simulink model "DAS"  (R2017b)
settings: Solver=FixedStepDiscrete  StartTime=0.0  StopTime=10.0  FixedStep=0.01  RelTol=1e-3  EnableMultiTasking=on
undefined symbols (not defined in the file): CcDAS_ACModeCurtLim_A, CcDAS_ACModeCurtTiLim_ms, CcDAS_BMSOperationConfirmTi_ms, CcDAS_CellMaxTempLim1_C, CcDAS_CellMaxTempLim2_C, CcDAS_CellMaxTempLim3_C, CcDAS_CellMaxTempLim4_C, CcDAS_CellMinTempHiLim_C, CcDAS_CellMinTempLowLim_C, CcDAS_CellMinTempMidLim_C, CcDAS_CellTempDiffLim_C, CcDAS_DCModeCurtTiLim_ms, CcDAS_HVSafetyNVMStoreTi_ms, CcDAS_OCVSOCDiffLim1_numb, CcDAS_OCVSOCDiffLim2_numb, CcDAS_PackCurrLim_A, CcDAS_SOCHighLim_numb, CcDAS_SOCLowerLim_numb, CcDAS_SOHLowerLim_numb, CcDAS_SOHLowerLimSale_numb, DAS_MIN2MS_NUMB, DAS_RUNTIME100_MS, DAS_RUNTIME10_MS, DAS_STATSTIMEMAX_MIN, DAS_STATSTIMEMIN_MIN, DAS_STATSTIMESMAX_NUMB, DAS_STATSTIMESMIN_NUMB, DAS_TIMESONE_NUMB, Enum_CTCCtrCtlConnMode
libraries: AIWAYS_Powertrain_BMS_lib x268
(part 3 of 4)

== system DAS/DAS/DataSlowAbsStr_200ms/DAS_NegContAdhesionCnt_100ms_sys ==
  GbISP_TFNegCloseFlt_flg : Inport
  EdgeRising : AIWAYS_Powertrain_BMS_lib/Logical Operators/EdgeRising
  TimesAddition : Subsystem  TreatAsAtomicUnit=on
  GcDAS_NegContAdhesionCnt_numb : Outport
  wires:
  GbISP_TFNegCloseFlt_flg/1 -> EdgeRising/1
  EdgeRising/1 -> TimesAddition/Enable
  TimesAddition/1(GcDAS_NegContAdhesionCnt_numb) -> GcDAS_NegContAdhesionCnt_numb/1

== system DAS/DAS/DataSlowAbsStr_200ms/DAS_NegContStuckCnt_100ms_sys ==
  GbISP_TFNegOpenFlt_flg : Inport
  EdgeRising : AIWAYS_Powertrain_BMS_lib/Logical Operators/EdgeRising
  TimesAddition : Subsystem  TreatAsAtomicUnit=on
  GcDAS_NegContStuckCnt_numb : Outport
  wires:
  GbISP_TFNegOpenFlt_flg/1 -> EdgeRising/1
  EdgeRising/1 -> TimesAddition/Enable
  TimesAddition/1(GcDAS_NegContStuckCnt_numb) -> GcDAS_NegContStuckCnt_numb/1

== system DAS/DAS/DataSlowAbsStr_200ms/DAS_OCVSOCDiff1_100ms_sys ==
  GcSOC_MaxCellSOC_pct : Inport
  GcSOC_MinCellSOC_pct : Inport  Port=2
  Comparison1 : RelationalOperator  OutDataTypeStr=boolean
  Comparison3 : RelationalOperator  Operator=>  OutDataTypeStr=boolean
  Constant1 : Constant  Value=CcDAS_OCVSOCDiffLim1_numb
  Constant2 : Constant  Value=CcDAS_OCVSOCDiffLim2_numb
  Logical : Logic  OutDataTypeStr=boolean
  OperationTimeCalc : Subsystem
  Sum1 : Sum  Inputs=+-  OutDataTypeStr=Inherit: Inherit via back propagation  RndMeth=Zero
  GcDAS_OCVSOCDiffTi1_min : Outport
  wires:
  OperationTimeCalc/1(GcDAS_OCVSOCDiffTi1_min) -> GcDAS_OCVSOCDiffTi1_min/1
  GcSOC_MaxCellSOC_pct/1 -> Sum1/1
  GcSOC_MinCellSOC_pct/1 -> Sum1/2
  Sum1/1 -> Comparison1/2, Comparison3/1
  Constant1/1 -> Comparison3/2
  Constant2/1 -> Comparison1/1
  Comparison1/1 -> Logical/1
  Comparison3/1 -> Logical/2
  Logical/1 -> OperationTimeCalc/Enable

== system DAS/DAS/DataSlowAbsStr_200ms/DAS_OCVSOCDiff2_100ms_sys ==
  GcSOC_MaxCellSOC_pct : Inport
  GcSOC_MinCellSOC_pct : Inport  Port=2
  Comparison3 : RelationalOperator  Operator=>  OutDataTypeStr=boolean
  Constant1 : Constant  Value=CcDAS_OCVSOCDiffLim2_numb
  OperationTimeCalc : Subsystem
  Sum1 : Sum  Inputs=+-  OutDataTypeStr=Inherit: Inherit via back propagation  RndMeth=Zero
  GcDAS_OCVSOCDiffTi2_min : Outport
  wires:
  OperationTimeCalc/1(GcDAS_OCVSOCDiffTi2_min) -> GcDAS_OCVSOCDiffTi2_min/1
  GcSOC_MaxCellSOC_pct/1 -> Sum1/1
  GcSOC_MinCellSOC_pct/1 -> Sum1/2
  Sum1/1 -> Comparison3/1
  Constant1/1 -> Comparison3/2
  Comparison3/1 -> OperationTimeCalc/Enable

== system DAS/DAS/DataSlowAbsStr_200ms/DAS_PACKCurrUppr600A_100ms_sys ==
  GbISP_TFPackCrntSaf_flg : Inport
  EdgeRising : AIWAYS_Powertrain_BMS_lib/Logical Operators/EdgeRising
  TimesAddition : Subsystem  TreatAsAtomicUnit=on
  GcDAS_TFPackCrntSafCnt_numb : Outport
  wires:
  GbISP_TFPackCrntSaf_flg/1 -> EdgeRising/1
  EdgeRising/1 -> TimesAddition/Enable
  TimesAddition/1(GcDAS_TFPackCrntSafCnt_numb) -> GcDAS_TFPackCrntSafCnt_numb/1

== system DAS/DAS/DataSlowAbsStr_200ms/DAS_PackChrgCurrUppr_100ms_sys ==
  GbISP_TFChrgPwrFltLevel3_flg : Inport
  EdgeRising : AIWAYS_Powertrain_BMS_lib/Logical Operators/EdgeRising
  TimesAddition : Subsystem  TreatAsAtomicUnit=on
  GcDAS_PackChrgCurrUpprLimCnt_numb : Outport
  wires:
  GbISP_TFChrgPwrFltLevel3_flg/1 -> EdgeRising/1
  EdgeRising/1 -> TimesAddition/Enable
  TimesAddition/1(GcDAS_PackChrgCurrUpprLimCnt_numb) -> GcDAS_PackChrgCurrUpprLimCnt_numb/1

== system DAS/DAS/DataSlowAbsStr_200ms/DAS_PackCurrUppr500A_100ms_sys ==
  GcHDP_PackCrnt_A : Inport
  Abs : Abs
  Comparison3 : RelationalOperator  OutDataTypeStr=boolean
  Constant4 : Constant  Value=CcDAS_PackCurrLim_A  OutDataTypeStr=single
  EdgeRising : AIWAYS_Powertrain_BMS_lib/Logical Operators/EdgeRising
  TimesAddition : Subsystem  TreatAsAtomicUnit=on
  GcDAS_PackCurrLim500ACnt_numb : Outport
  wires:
  GcHDP_PackCrnt_A/1 -> Abs/1
  EdgeRising/1 -> TimesAddition/Enable
  TimesAddition/1(GcDAS_PackCurrLim500ACnt_numb) -> GcDAS_PackCurrLim500ACnt_numb/1
  Comparison3/1 -> EdgeRising/1
  Constant4/1 -> Comparison3/2
  Abs/1 -> Comparison3/1

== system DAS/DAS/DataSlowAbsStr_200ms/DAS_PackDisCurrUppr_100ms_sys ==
  GbISP_TFDisChrgPwrFltLevel3_flg : Inport
  EdgeRising : AIWAYS_Powertrain_BMS_lib/Logical Operators/EdgeRising
  TimesAddition : Subsystem  TreatAsAtomicUnit=on
  GcDAS_PackDisCurrUpprLimCnt_numb : Outport
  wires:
  GbISP_TFDisChrgPwrFltLevel3_flg/1 -> EdgeRising/1
  EdgeRising/1 -> TimesAddition/Enable
  TimesAddition/1(GcDAS_PackDisCurrUpprLimCnt_numb) -> GcDAS_PackDisCurrUpprLimCnt_numb/1

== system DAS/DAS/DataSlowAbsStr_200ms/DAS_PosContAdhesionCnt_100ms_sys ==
  GbISP_TFPosCloseFlt_flg : Inport
  EdgeRising : AIWAYS_Powertrain_BMS_lib/Logical Operators/EdgeRising
  TimesAddition : Subsystem  TreatAsAtomicUnit=on
  GcDAS_PosContAdhesionCnt_numb : Outport
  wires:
  GbISP_TFPosCloseFlt_flg/1 -> EdgeRising/1
  EdgeRising/1 -> TimesAddition/Enable
  TimesAddition/1(GcDAS_PosContAdhesionCnt_numb) -> GcDAS_PosContAdhesionCnt_numb/1

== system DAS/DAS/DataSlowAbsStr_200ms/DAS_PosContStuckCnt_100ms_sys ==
  GbISP_TFPosOpenFlt_flg : Inport
  EdgeRising : AIWAYS_Powertrain_BMS_lib/Logical Operators/EdgeRising
  TimesAddition : Subsystem  TreatAsAtomicUnit=on
  GcDAS_PosContStuckCnt_numb : Outport
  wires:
  GbISP_TFPosOpenFlt_flg/1 -> EdgeRising/1
  EdgeRising/1 -> TimesAddition/Enable
  TimesAddition/1(GcDAS_PosContStuckCnt_numb) -> GcDAS_PosContStuckCnt_numb/1

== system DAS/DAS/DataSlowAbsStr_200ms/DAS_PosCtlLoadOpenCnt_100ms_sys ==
  GcISP_ShutDownPosCtlLoadOpen_flg : Inport
  EdgeRising : AIWAYS_Powertrain_BMS_lib/Logical Operators/EdgeRising
  TimesAddition : Subsystem  TreatAsAtomicUnit=on
  GcDAS_PosCtlLoadOpenCnt_numb : Outport
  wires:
  GcISP_ShutDownPosCtlLoadOpen_flg/1 -> EdgeRising/1
  TimesAddition/1(GcDAS_PosCtlLoadOpenCnt_numb) -> GcDAS_PosCtlLoadOpenCnt_numb/1
  EdgeRising/1 -> TimesAddition/Enable

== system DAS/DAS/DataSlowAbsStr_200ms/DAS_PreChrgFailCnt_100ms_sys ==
  GbISP_TFPreChrgFail_flg : Inport
  EdgeRising : AIWAYS_Powertrain_BMS_lib/Logical Operators/EdgeRising
  TimesAddition : Subsystem  TreatAsAtomicUnit=on
  GcDAS_PreChrgFailCnt_numb : Outport
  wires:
  GbISP_TFPreChrgFail_flg/1 -> EdgeRising/1
  EdgeRising/1 -> TimesAddition/Enable
  TimesAddition/1(GcDAS_PreChrgFailCnt_numb) -> GcDAS_PreChrgFailCnt_numb/1

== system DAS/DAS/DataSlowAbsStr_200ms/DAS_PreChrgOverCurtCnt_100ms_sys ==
  GbISP_TFPreChrgOverCurt_flg : Inport
  EdgeRising : AIWAYS_Powertrain_BMS_lib/Logical Operators/EdgeRising
  TimesAddition : Subsystem  TreatAsAtomicUnit=on
  GcDAS_PreChrgOvrCurrCnt_numb : Outport
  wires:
  GbISP_TFPreChrgOverCurt_flg/1 -> EdgeRising/1
  EdgeRising/1 -> TimesAddition/Enable
  TimesAddition/1(GcDAS_PreChrgOvrCurrCnt_numb) -> GcDAS_PreChrgOvrCurrCnt_numb/1

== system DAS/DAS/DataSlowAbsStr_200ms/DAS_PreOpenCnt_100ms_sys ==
  GbISP_TFPreOpenFlt_flg : Inport
  EdgeRising : AIWAYS_Powertrain_BMS_lib/Logical Operators/EdgeRising
  TimesAddition : Subsystem  TreatAsAtomicUnit=on
  GcDAS_PreChrgOpenCnt_numb : Outport
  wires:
  GbISP_TFPreOpenFlt_flg/1 -> EdgeRising/1
  EdgeRising/1 -> TimesAddition/Enable
  TimesAddition/1(GcDAS_PreChrgOpenCnt_numb) -> GcDAS_PreChrgOpenCnt_numb/1

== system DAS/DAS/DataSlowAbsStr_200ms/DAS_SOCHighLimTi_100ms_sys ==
  GcSOC_PackSOC_pct : Inport
  Comparison3 : RelationalOperator  OutDataTypeStr=boolean
  Constant7 : Constant  Value=CcDAS_SOCHighLim_numb
  Data Type Conversion : DataTypeConversion  OutDataTypeStr=single
  OperationTimeCalc : Subsystem
  GcDAS_SOCHighLimTi_min : Outport
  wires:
  GcSOC_PackSOC_pct/1 -> Comparison3/1
  Constant7/1 -> Data Type Conversion/1
  OperationTimeCalc/1(GcDAS_SOCHighLimTi_min) -> GcDAS_SOCHighLimTi_min/1
  Data Type Conversion/1 -> Comparison3/2
  Comparison3/1 -> OperationTimeCalc/Enable

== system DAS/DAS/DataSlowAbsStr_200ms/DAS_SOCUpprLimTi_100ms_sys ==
  GcSOC_PackSOC_pct : Inport
  Comparison3 : RelationalOperator  Operator=<=  OutDataTypeStr=boolean
  Constant7 : Constant  Value=CcDAS_SOCLowerLim_numb
  Data Type Conversion : DataTypeConversion  OutDataTypeStr=single
  OperationTimeCalc : Subsystem
  GcDAS_SOCLowLimTi_min : Outport
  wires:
  GcSOC_PackSOC_pct/1 -> Comparison3/1
  Constant7/1 -> Data Type Conversion/1
  OperationTimeCalc/1(GcDAS_SOCLowLimTi_min) -> GcDAS_SOCLowLimTi_min/1
  Data Type Conversion/1 -> Comparison3/2
  Comparison3/1 -> OperationTimeCalc/Enable

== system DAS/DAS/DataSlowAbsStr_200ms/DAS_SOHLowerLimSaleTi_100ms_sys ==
  GcSOH_PackSOH_pct : Inport
  Comparison3 : RelationalOperator  Operator=<=  OutDataTypeStr=boolean
  Constant7 : Constant  Value=CcDAS_SOHLowerLimSale_numb
  Data Type Conversion : DataTypeConversion  OutDataTypeStr=single
  OperationTimeCalc : Subsystem
  GcDAS_SOHLowerLimSaleTi_min : Outport
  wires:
  GcSOH_PackSOH_pct/1 -> Comparison3/1
  Constant7/1 -> Data Type Conversion/1
  Comparison3/1 -> OperationTimeCalc/Enable
  OperationTimeCalc/1(GcDAS_SOHLowerLimSaleTi_min) -> GcDAS_SOHLowerLimSaleTi_min/1
  Data Type Conversion/1 -> Comparison3/2

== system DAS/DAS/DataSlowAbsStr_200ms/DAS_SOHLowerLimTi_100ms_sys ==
  GcSOH_PackSOH_pct : Inport
  Comparison3 : RelationalOperator  Operator=<=  OutDataTypeStr=boolean
  Constant7 : Constant  Value=CcDAS_SOHLowerLim_numb
  Data Type Conversion : DataTypeConversion  OutDataTypeStr=single
  OperationTimeCalc : Subsystem
  GcDAS_SOHLowerLimTi_min : Outport
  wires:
  GcSOH_PackSOH_pct/1 -> Comparison3/1
  Constant7/1 -> Data Type Conversion/1
  Comparison3/1 -> OperationTimeCalc/Enable
  OperationTimeCalc/1(GcDAS_SOHLowerLimTi_min) -> GcDAS_SOHLowerLimTi_min/1
  Data Type Conversion/1 -> Comparison3/2

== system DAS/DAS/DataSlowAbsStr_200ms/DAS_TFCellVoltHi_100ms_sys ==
  GbISP_TFHighCellVoltSaf_flg : Inport
  EdgeRising : AIWAYS_Powertrain_BMS_lib/Logical Operators/EdgeRising
  TimesAddition : Subsystem  TreatAsAtomicUnit=on
  GcDAS_CellVoltUpprLimCnt_numb : Outport
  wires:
  GbISP_TFHighCellVoltSaf_flg/1 -> EdgeRising/1
  EdgeRising/1 -> TimesAddition/Enable
  TimesAddition/1(GcDAS_CellVoltUpprLimCnt_numb) -> GcDAS_CellVoltUpprLimCnt_numb/1

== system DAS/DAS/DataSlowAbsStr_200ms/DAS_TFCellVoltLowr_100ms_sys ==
  GbISP_TFLowCellVoltSaf_flg : Inport
  EdgeRising : AIWAYS_Powertrain_BMS_lib/Logical Operators/EdgeRising
  TimesAddition : Subsystem  TreatAsAtomicUnit=on
  GcDAS_CellVoltLowrLimCnt_numb : Outport
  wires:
  GbISP_TFLowCellVoltSaf_flg/1 -> EdgeRising/1
  EdgeRising/1 -> TimesAddition/Enable
  TimesAddition/1(GcDAS_CellVoltLowrLimCnt_numb) -> GcDAS_CellVoltLowrLimCnt_numb/1

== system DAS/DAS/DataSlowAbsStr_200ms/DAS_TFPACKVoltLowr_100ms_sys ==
  GbISP_TFPackVoltHiAlrmFlt_flg : Inport
  EdgeRising : AIWAYS_Powertrain_BMS_lib/Logical Operators/EdgeRising
  TimesAddition : Subsystem  TreatAsAtomicUnit=on
  GcDAS_BattVoltUpprLimCnt_numb : Outport
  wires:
  GbISP_TFPackVoltHiAlrmFlt_flg/1 -> EdgeRising/1
  EdgeRising/1 -> TimesAddition/Enable
  TimesAddition/1(GcDAS_BattVoltUpprLimCnt_numb) -> GcDAS_BattVoltUpprLimCnt_numb/1

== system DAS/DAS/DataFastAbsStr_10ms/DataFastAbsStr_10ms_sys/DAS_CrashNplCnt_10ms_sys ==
  GbISP_TFCANCrashFlt_flg : Inport
  GbISP_TFHWCrashFlt_flg : Inport  Port=2
  EdgeRising : AIWAYS_Powertrain_BMS_lib/Logical Operators/EdgeRising
  Logical1 : Logic  Operator=OR  OutDataTypeStr=boolean
  TimesAddition : Subsystem  TreatAsAtomicUnit=on
  GcDAS_CrashNplCnt_numb : Outport
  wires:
  EdgeRising/1 -> TimesAddition/Enable
  TimesAddition/1(GcDAS_CrashNplCnt_numb) -> GcDAS_CrashNplCnt_numb/1
  GbISP_TFCANCrashFlt_flg/1 -> Logical1/1
  GbISP_TFHWCrashFlt_flg/1 -> Logical1/2
  Logical1/1 -> EdgeRising/1

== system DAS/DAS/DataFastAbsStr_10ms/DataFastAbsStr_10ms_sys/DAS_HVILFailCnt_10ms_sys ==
  GbISP_TFHvilLFlt_flg : Inport
  GbISP_TFHvilSTG_flg : Inport  Port=2
  GbISP_TFHvilSTV_flg : Inport  Port=3
  EdgeRising : AIWAYS_Powertrain_BMS_lib/Logical Operators/EdgeRising
  Logical1 : Logic  Operator=OR  Inputs=3  OutDataTypeStr=boolean
  TimesAddition : Subsystem  TreatAsAtomicUnit=on
  GcDAS_HVILFailCnt_numb : Outport
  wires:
  EdgeRising/1 -> TimesAddition/Enable
  TimesAddition/1(GcDAS_HVILFailCnt_numb) -> GcDAS_HVILFailCnt_numb/1
  GbISP_TFHvilLFlt_flg/1 -> Logical1/1
  Logical1/1 -> EdgeRising/1
  GbISP_TFHvilSTG_flg/1 -> Logical1/2
  GbISP_TFHvilSTV_flg/1 -> Logical1/3

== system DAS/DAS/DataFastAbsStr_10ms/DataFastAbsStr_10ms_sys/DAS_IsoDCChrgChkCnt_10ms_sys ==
  GbISP_TFIsoDCResFltLevel1_flg : Inport
  GbISP_TFIsoDCResFltLevel2_flg : Inport  Port=2
  EdgeRising : AIWAYS_Powertrain_BMS_lib/Logical Operators/EdgeRising
  Logical1 : Logic  Operator=OR  OutDataTypeStr=boolean
  TimesAddition : Subsystem  TreatAsAtomicUnit=on
  GcDAS_IsoDCChrgChkCnt_numb : Outport
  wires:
  EdgeRising/1 -> TimesAddition/Enable
  TimesAddition/1(GcDAS_IsoDCChrgChkCnt_numb) -> GcDAS_IsoDCChrgChkCnt_numb/1
  GbISP_TFIsoDCResFltLevel1_flg/1 -> Logical1/1
  Logical1/1 -> EdgeRising/1
  GbISP_TFIsoDCResFltLevel2_flg/1 -> Logical1/2

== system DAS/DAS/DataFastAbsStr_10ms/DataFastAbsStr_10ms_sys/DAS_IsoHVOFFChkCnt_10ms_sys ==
  GbISP_TFIsoHVoffResFltLevel1_flg : Inport
  GbISP_TFIsoHVoffResFltLevel2_flg : Inport  Port=2
  EdgeRising : AIWAYS_Powertrain_BMS_lib/Logical Operators/EdgeRising
  Logical1 : Logic  Operator=OR  OutDataTypeStr=boolean
  TimesAddition : Subsystem  TreatAsAtomicUnit=on
  GcDAS_IsoHVOFFChkCnt_numb : Outport
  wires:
  EdgeRising/1 -> TimesAddition/Enable
  TimesAddition/1(GcDAS_IsoHVOFFChkCnt_numb) -> GcDAS_IsoHVOFFChkCnt_numb/1
  GbISP_TFIsoHVoffResFltLevel1_flg/1 -> Logical1/1
  Logical1/1 -> EdgeRising/1
  GbISP_TFIsoHVoffResFltLevel2_flg/1 -> Logical1/2

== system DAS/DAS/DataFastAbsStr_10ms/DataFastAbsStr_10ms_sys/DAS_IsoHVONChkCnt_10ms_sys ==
  GbISP_TFIsoResFltLevel1_flg : Inport
  GbISP_TFIsoResFltLevel2_flg : Inport  Port=2
  EdgeRising : AIWAYS_Powertrain_BMS_lib/Logical Operators/EdgeRising
  Logical1 : Logic  Operator=OR  OutDataTypeStr=boolean
  TimesAddition : Subsystem  TreatAsAtomicUnit=on
  GcDAS_IsoHVONChkCnt_numb : Outport
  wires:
  EdgeRising/1 -> TimesAddition/Enable
  TimesAddition/1(GcDAS_IsoHVONChkCnt_numb) -> GcDAS_IsoHVONChkCnt_numb/1
  GbISP_TFIsoResFltLevel1_flg/1 -> Logical1/1
  Logical1/1 -> EdgeRising/1
  GbISP_TFIsoResFltLevel2_flg/1 -> Logical1/2

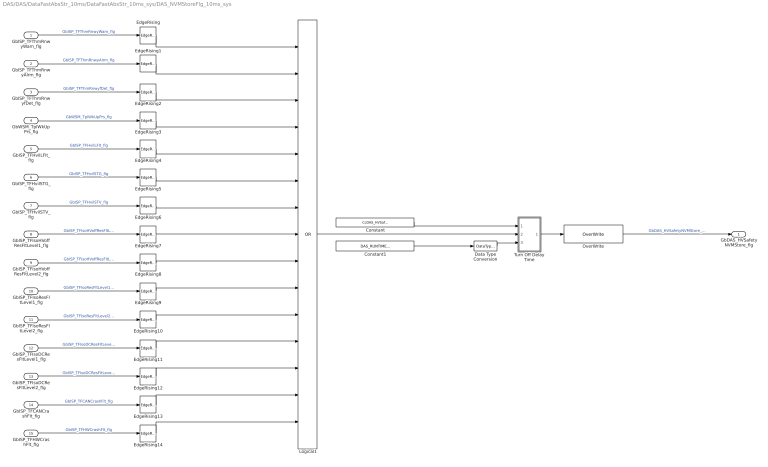
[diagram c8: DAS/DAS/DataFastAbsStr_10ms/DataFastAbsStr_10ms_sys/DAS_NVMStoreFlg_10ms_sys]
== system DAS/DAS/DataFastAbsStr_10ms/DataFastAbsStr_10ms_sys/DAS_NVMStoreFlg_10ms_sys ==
  GbISP_TFThmRnwyWarn_flg : Inport
  GbISP_TFThmRnwyAlrm_flg : Inport  Port=2
  GbISP_TFThmRnwyfDet_flg : Inport  Port=3
  GbWSM_TplWkUpPrs_flg : Inport  Port=4
  GbISP_TFHvilLFlt_flg : Inport  Port=5
  GbISP_TFHvilSTG_flg : Inport  Port=6
  GbISP_TFHvilSTV_flg : Inport  Port=7
  GbISP_TFIsoHVoffResFltLevel1_flg : Inport  Port=8
  GbISP_TFIsoHVoffResFltLevel2_flg : Inport  Port=9
  GbISP_TFIsoResFltLevel1_flg : Inport  Port=10
  GbISP_TFIsoResFltLevel2_flg : Inport  Port=11
  GbISP_TFIsoDCResFltLevel1_flg : Inport  Port=12
  GbISP_TFIsoDCResFltLevel2_flg : Inport  Port=13
  GbISP_TFCANCrashFlt_flg : Inport  Port=14
  GbISP_TFHWCrashFlt_flg : Inport  Port=15
  Constant : Constant  Value=CcDAS_HVSafetyNVMStoreTi_ms
  Constant1 : Constant  Value=DAS_RUNTIME10_MS
  Data Type Conversion : DataTypeConversion  OutDataTypeStr=uint16
  EdgeRising{,1..14} (15 alike) : AIWAYS_Powertrain_BMS_lib/Logical Operators/EdgeRising
  Logical1 : Logic  Operator=OR  Inputs=15  OutDataTypeStr=boolean
  OverWrite : AIWAYS_Powertrain_BMS_lib/Signals/OverWrite  OverWrite_Value=CbDAS_HVSafetyNVMStoreOvr_flg  OverWrite_flag=CbDAS_HVSafetyNVMStoreOvrSwt_flg
  Turn Off Delay Time : Subsystem  TreatAsAtomicUnit=on  mask(TurnOffDelayTime){}
      mask help: The falling edge of the input signal (u) is delayed by the input delay time (T). Input1= Delay Time; Input2=Signal (u); Input3=Activation Rate.
  GbDAS_HVSafetyNVMStore_flg : Outport
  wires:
  GbISP_TFThmRnwyWarn_flg/1 -> EdgeRising/1  "GbISP_TFThmRnwyWarn_flg"
  GbISP_TFThmRnwyAlrm_flg/1 -> EdgeRising1/1  "GbISP_TFThmRnwyAlrm_flg"
  GbISP_TFThmRnwyfDet_flg/1 -> EdgeRising2/1  "GbISP_TFThmRnwyfDet_flg"
  GbWSM_TplWkUpPrs_flg/1 -> EdgeRising3/1  "GbWSM_TplWkUpPrs_flg"
  GbISP_TFHvilLFlt_flg/1 -> EdgeRising4/1  "GbISP_TFHvilLFlt_flg"
  GbISP_TFHvilSTG_flg/1 -> EdgeRising5/1  "GbISP_TFHvilSTG_flg"
  GbISP_TFHvilSTV_flg/1 -> EdgeRising6/1  "GbISP_TFHvilSTV_flg"
  GbISP_TFIsoHVoffResFltLevel1_flg/1 -> EdgeRising7/1  "GbISP_TFIsoHVoffResFltLevel1_flg"
  GbISP_TFIsoHVoffResFltLevel2_flg/1 -> EdgeRising8/1  "GbISP_TFIsoHVoffResFltLevel2_flg"
  GbISP_TFIsoResFltLevel1_flg/1 -> EdgeRising9/1  "GbISP_TFIsoResFltLevel1_flg"
  GbISP_TFIsoResFltLevel2_flg/1 -> EdgeRising10/1  "GbISP_TFIsoResFltLevel2_flg"
  GbISP_TFIsoDCResFltLevel1_flg/1 -> EdgeRising11/1  "GbISP_TFIsoDCResFltLevel1_flg"
  GbISP_TFIsoDCResFltLevel2_flg/1 -> EdgeRising12/1  "GbISP_TFIsoDCResFltLevel2_flg"
  GbISP_TFCANCrashFlt_flg/1 -> EdgeRising13/1  "GbISP_TFCANCrashFlt_flg"
  GbISP_TFHWCrashFlt_flg/1 -> EdgeRising14/1  "GbISP_TFHWCrashFlt_flg"
  Turn Off Delay Time/1(y) -> OverWrite/1
  EdgeRising/1 -> Logical1/1
  EdgeRising1/1 -> Logical1/2
  EdgeRising2/1 -> Logical1/3
  EdgeRising3/1 -> Logical1/4
  EdgeRising4/1 -> Logical1/5
  EdgeRising5/1 -> Logical1/6
  EdgeRising6/1 -> Logical1/7
  EdgeRising7/1 -> Logical1/8
  EdgeRising8/1 -> Logical1/9
  EdgeRising9/1 -> Logical1/10
  EdgeRising10/1 -> Logical1/11
  EdgeRising11/1 -> Logical1/12
  EdgeRising12/1 -> Logical1/13
  EdgeRising13/1 -> Logical1/14
  EdgeRising14/1 -> Logical1/15
  Logical1/1 -> Turn Off Delay Time/2(u)
  Constant/1 -> Turn Off Delay Time/1(T)
  Constant1/1 -> Data Type Conversion/1
  OverWrite/1 -> GbDAS_HVSafetyNVMStore_flg/1  "GbDAS_HVSafetyNVMStore_flg"
  Data Type Conversion/1 -> Turn Off Delay Time/3(dT)

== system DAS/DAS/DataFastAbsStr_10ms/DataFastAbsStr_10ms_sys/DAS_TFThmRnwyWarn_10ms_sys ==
  GbISP_TFThmRnwyWarn_flg : Inport
  EdgeRising : AIWAYS_Powertrain_BMS_lib/Logical Operators/EdgeRising
  TimesAddition : Subsystem  TreatAsAtomicUnit=on
  GcDAS_ThmRnwyWarnCnt_numb : Outport
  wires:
  EdgeRising/1 -> TimesAddition/Enable
  TimesAddition/1(GcDAS_ThmRnwyWarnCnt_numb) -> GcDAS_ThmRnwyWarnCnt_numb/1
  GbISP_TFThmRnwyWarn_flg/1 -> EdgeRising/1

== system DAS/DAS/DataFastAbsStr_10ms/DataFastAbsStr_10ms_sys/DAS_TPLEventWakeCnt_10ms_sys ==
  GbWSM_TplWkUpPrs_flg : Inport
  EdgeRising : AIWAYS_Powertrain_BMS_lib/Logical Operators/EdgeRising
  TimesAddition : Subsystem  TreatAsAtomicUnit=on
  GcDAS_TPLEventWakeCnt_numb : Outport
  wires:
  EdgeRising/1 -> TimesAddition/Enable
  TimesAddition/1(GcDAS_TPLEventWakeCnt_numb) -> GcDAS_TPLEventWakeCnt_numb/1
  GbWSM_TplWkUpPrs_flg/1 -> EdgeRising/1

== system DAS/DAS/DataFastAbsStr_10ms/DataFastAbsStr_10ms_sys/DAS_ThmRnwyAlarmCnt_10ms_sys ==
  GbISP_TFThmRnwyAlrm_flg : Inport
  EdgeRising : AIWAYS_Powertrain_BMS_lib/Logical Operators/EdgeRising
  TimesAddition : Subsystem  TreatAsAtomicUnit=on
  GcDAS_ThmRnwyAlarmCnt_numb : Outport
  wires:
  EdgeRising/1 -> TimesAddition/Enable
  TimesAddition/1(GcDAS_ThmRnwyAlarmCnt_numb) -> GcDAS_ThmRnwyAlarmCnt_numb/1
  GbISP_TFThmRnwyAlrm_flg/1 -> EdgeRising/1

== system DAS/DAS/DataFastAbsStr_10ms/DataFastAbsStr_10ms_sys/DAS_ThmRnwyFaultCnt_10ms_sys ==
  GbISP_TFThmRnwyfDet_flg : Inport
  EdgeRising : AIWAYS_Powertrain_BMS_lib/Logical Operators/EdgeRising
  TimesAddition : Subsystem  TreatAsAtomicUnit=on
  GcDAS_ThmRnwyFaultCnt_numb : Outport
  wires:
  EdgeRising/1 -> TimesAddition/Enable
  TimesAddition/1(GcDAS_ThmRnwyFaultCnt_numb) -> GcDAS_ThmRnwyFaultCnt_numb/1
  GbISP_TFThmRnwyfDet_flg/1 -> EdgeRising/1

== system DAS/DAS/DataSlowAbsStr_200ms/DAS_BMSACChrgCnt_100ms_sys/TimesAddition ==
  Enable : EnablePort
  ACC_GbACC_ACChrgMismatch_flg : AIWAYS_Powertrain_BMS_lib/Signals/OverWrite  OverWrite_Value=CcDAS_BMSACChrgCntOvr_numb  OverWrite_flag=CbDAS_BMSACChrgCntOvrSwt_flg
  Constant : Constant  Value=DAS_TIMESONE_NUMB
  Constant4 : Constant  Value=DAS_STATSTIMESMIN_NUMB
  Constant5 : Constant  Value=DAS_STATSTIMESMAX_NUMB
  Data Store Read : AIWAYS_Powertrain_BMS_lib/Signals/Data Store Read  Priority=0  DSR=EcNVM_BMSACChrgCnt_numb
  Data Store Write : AIWAYS_Powertrain_BMS_lib/Signals/Data Store Write  DSW=EcNVM_BMSACChrgCnt_numb
  Data Type Conversion : DataTypeConversion  OutDataTypeStr=single
  Limiter : AIWAYS_Powertrain_BMS_lib/Nonlinear Blocks/Limiter
  Sum : Sum  OutDataTypeStr=Inherit: Inherit via back propagation  RndMeth=Zero
  GcDAS_BMSACChrgCnt_numb : Outport
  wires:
  Data Store Read/1 -> Sum/1
  Sum/1 -> Limiter/3
  ACC_GbACC_ACChrgMismatch_flg/1 -> GcDAS_BMSACChrgCnt_numb/1, Data Store Write/1  "GcDAS_BMSACChrgCnt_numb"
  Constant/1 -> Data Type Conversion/1
  Constant5/1 -> Limiter/1
  Constant4/1 -> Limiter/2
  Limiter/1 -> ACC_GbACC_ACChrgMismatch_flg/1
  Data Type Conversion/1 -> Sum/2

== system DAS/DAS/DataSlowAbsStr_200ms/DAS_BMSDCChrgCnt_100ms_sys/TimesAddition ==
  Enable : EnablePort
  ACC_GbACC_ACChrgMismatch_flg : AIWAYS_Powertrain_BMS_lib/Signals/OverWrite  OverWrite_Value=CcDAS_BMSDCChrgCntOvr_numb  OverWrite_flag=CbDAS_BMSDCChrgCntOvrSwt_flg
  Constant : Constant  Value=DAS_TIMESONE_NUMB
  Constant4 : Constant  Value=DAS_STATSTIMESMIN_NUMB
  Constant5 : Constant  Value=DAS_STATSTIMESMAX_NUMB
  Data Store Read : AIWAYS_Powertrain_BMS_lib/Signals/Data Store Read  Priority=0  DSR=EcNVM_BMSDCChrgCnt_numb
  Data Store Write : AIWAYS_Powertrain_BMS_lib/Signals/Data Store Write  DSW=EcNVM_BMSDCChrgCnt_numb
  Limiter : AIWAYS_Powertrain_BMS_lib/Nonlinear Blocks/Limiter
  Sum : Sum  OutDataTypeStr=Inherit: Inherit via back propagation  RndMeth=Zero
  GcDAS_BMSDCChrgCnt_numb : Outport
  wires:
  Data Store Read/1 -> Sum/1
  Sum/1 -> Limiter/3
  ACC_GbACC_ACChrgMismatch_flg/1 -> GcDAS_BMSDCChrgCnt_numb/1, Data Store Write/1  "GcDAS_BMSDCChrgCnt_numb"
  Constant5/1 -> Limiter/1
  Constant4/1 -> Limiter/2
  Limiter/1 -> ACC_GbACC_ACChrgMismatch_flg/1
  Constant/1 -> Sum/2

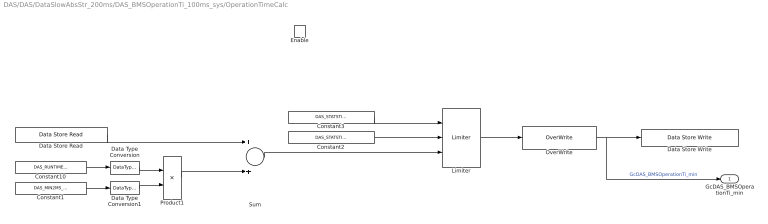
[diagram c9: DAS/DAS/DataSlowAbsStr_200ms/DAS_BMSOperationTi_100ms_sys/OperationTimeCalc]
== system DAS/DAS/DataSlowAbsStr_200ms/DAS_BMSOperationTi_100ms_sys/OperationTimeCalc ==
  Enable : EnablePort
  Constant1 : Constant  Value=DAS_MIN2MS_NUMB
  Constant10 : Constant  Value=DAS_RUNTIME100_MS
  Constant2 : Constant  Value=DAS_STATSTIMEMIN_MIN
  Constant3 : Constant  Value=DAS_STATSTIMEMAX_MIN
  Data Store Read : AIWAYS_Powertrain_BMS_lib/Signals/Data Store Read  Priority=0  DSR=EcNVM_BMSOperationTi_min
  Data Store Write : AIWAYS_Powertrain_BMS_lib/Signals/Data Store Write  DSW=EcNVM_BMSOperationTi_min
  Data Type Conversion : DataTypeConversion  OutDataTypeStr=single
  Data Type Conversion1 : DataTypeConversion  OutDataTypeStr=single
  Limiter : AIWAYS_Powertrain_BMS_lib/Nonlinear Blocks/Limiter
  OverWrite : AIWAYS_Powertrain_BMS_lib/Signals/OverWrite  OverWrite_Value=CcDAS_BMSOperationTiOvr_min  OverWrite_flag=CbDAS_BMSOperationTiOvrSwt_flg
  Product1 : Product  Inputs=*/  OutDataTypeStr=Inherit: Inherit via back propagation
  Sum : Sum  OutDataTypeStr=Inherit: Inherit via back propagation  RndMeth=Zero
  GcDAS_BMSOperationTi_min : Outport
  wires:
  Data Store Read/1 -> Sum/1
  Constant10/1 -> Data Type Conversion/1
  Data Type Conversion/1 -> Product1/1
  Product1/1 -> Sum/2
  Constant1/1 -> Data Type Conversion1/1
  Data Type Conversion1/1 -> Product1/2
  Sum/1 -> Limiter/3
  Limiter/1 -> OverWrite/1
  Constant2/1 -> Limiter/2
  Constant3/1 -> Limiter/1
  OverWrite/1 -> Data Store Write/1, GcDAS_BMSOperationTi_min/1  "GcDAS_BMSOperationTi_min"

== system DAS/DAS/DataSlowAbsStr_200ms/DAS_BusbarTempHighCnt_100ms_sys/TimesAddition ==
  Enable : EnablePort
  ACC_GbACC_ACChrgMismatch_flg : AIWAYS_Powertrain_BMS_lib/Signals/OverWrite  OverWrite_Value=CcDAS_BusbarTempHighCntOvr_numb  OverWrite_flag=CbDAS_BusbarTempHighCntOvrSwt_flg
  Constant : Constant  Value=DAS_TIMESONE_NUMB
  Constant4 : Constant  Value=DAS_STATSTIMESMIN_NUMB
  Constant5 : Constant  Value=DAS_STATSTIMESMAX_NUMB
  Data Store Read : AIWAYS_Powertrain_BMS_lib/Signals/Data Store Read  Priority=0  DSR=EcNVM_BusbarTempHighCnt_numb
  Data Store Write : AIWAYS_Powertrain_BMS_lib/Signals/Data Store Write  DSW=EcNVM_BusbarTempHighCnt_numb
  Limiter : AIWAYS_Powertrain_BMS_lib/Nonlinear Blocks/Limiter
  Sum : Sum  OutDataTypeStr=Inherit: Inherit via back propagation  RndMeth=Zero
  GcDAS_BusbarTempHighCnt_numb : Outport
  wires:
  Data Store Read/1 -> Sum/1
  Sum/1 -> Limiter/3
  ACC_GbACC_ACChrgMismatch_flg/1 -> GcDAS_BusbarTempHighCnt_numb/1, Data Store Write/1  "GcDAS_BusbarTempHighCnt_numb"
  Constant/1 -> Sum/2
  Constant5/1 -> Limiter/1
  Constant4/1 -> Limiter/2
  Limiter/1 -> ACC_GbACC_ACChrgMismatch_flg/1

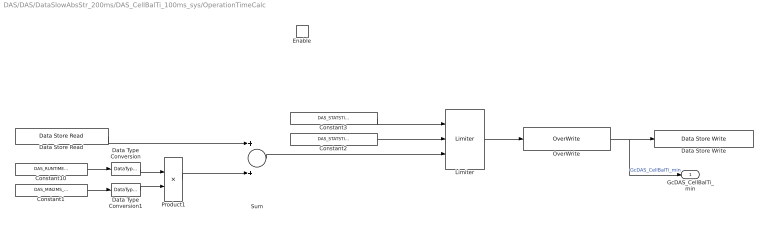
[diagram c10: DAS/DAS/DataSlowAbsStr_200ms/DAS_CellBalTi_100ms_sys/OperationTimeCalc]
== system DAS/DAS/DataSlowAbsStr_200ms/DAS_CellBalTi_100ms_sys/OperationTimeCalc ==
  Enable : EnablePort
  Constant1 : Constant  Value=DAS_MIN2MS_NUMB
  Constant10 : Constant  Value=DAS_RUNTIME100_MS
  Constant2 : Constant  Value=DAS_STATSTIMEMIN_MIN
  Constant3 : Constant  Value=DAS_STATSTIMEMAX_MIN
  Data Store Read : AIWAYS_Powertrain_BMS_lib/Signals/Data Store Read  Priority=0  DSR=EcNVM_CellBalTi_min
  Data Store Write : AIWAYS_Powertrain_BMS_lib/Signals/Data Store Write  DSW=EcNVM_CellBalTi_min
  Data Type Conversion : DataTypeConversion  OutDataTypeStr=single
  Data Type Conversion1 : DataTypeConversion  OutDataTypeStr=single
  Limiter : AIWAYS_Powertrain_BMS_lib/Nonlinear Blocks/Limiter
  OverWrite : AIWAYS_Powertrain_BMS_lib/Signals/OverWrite  OverWrite_Value=CcDAS_CellBalTiOvr_min  OverWrite_flag=CbDAS_CellBalTiOvrSwt_flg
  Product1 : Product  Inputs=*/  OutDataTypeStr=Inherit: Inherit via back propagation
  Sum : Sum  OutDataTypeStr=Inherit: Inherit via back propagation  RndMeth=Zero
  GcDAS_CellBalTi_min : Outport
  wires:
  Data Store Read/1 -> Sum/1
  Constant10/1 -> Data Type Conversion/1
  Data Type Conversion/1 -> Product1/1
  Product1/1 -> Sum/2
  Constant1/1 -> Data Type Conversion1/1
  Data Type Conversion1/1 -> Product1/2
  Sum/1 -> Limiter/3
  Limiter/1 -> OverWrite/1
  Constant2/1 -> Limiter/2
  Constant3/1 -> Limiter/1
  OverWrite/1 -> Data Store Write/1, GcDAS_CellBalTi_min/1  "GcDAS_CellBalTi_min"

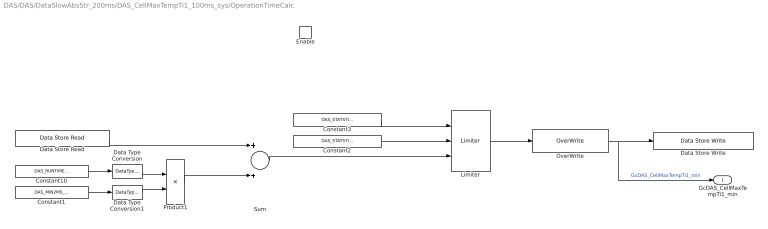
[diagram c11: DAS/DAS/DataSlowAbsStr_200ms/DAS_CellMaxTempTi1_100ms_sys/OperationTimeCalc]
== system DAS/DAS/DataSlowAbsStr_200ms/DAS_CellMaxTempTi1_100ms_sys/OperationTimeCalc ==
  Enable : EnablePort
  Constant1 : Constant  Value=DAS_MIN2MS_NUMB
  Constant10 : Constant  Value=DAS_RUNTIME100_MS
  Constant2 : Constant  Value=DAS_STATSTIMEMIN_MIN
  Constant3 : Constant  Value=DAS_STATSTIMEMAX_MIN
  Data Store Read : AIWAYS_Powertrain_BMS_lib/Signals/Data Store Read  Priority=0  DSR=EcNVM_CellMaxTempTi1_min
  Data Store Write : AIWAYS_Powertrain_BMS_lib/Signals/Data Store Write  DSW=EcNVM_CellMaxTempTi1_min
  Data Type Conversion : DataTypeConversion  OutDataTypeStr=single
  Data Type Conversion1 : DataTypeConversion  OutDataTypeStr=single
  Limiter : AIWAYS_Powertrain_BMS_lib/Nonlinear Blocks/Limiter
  OverWrite : AIWAYS_Powertrain_BMS_lib/Signals/OverWrite  OverWrite_Value=CcDAS_CellMaxTempTi1Ovr_min  OverWrite_flag=CbDAS_CellMaxTempTi1OvrSwt_flg
  Product1 : Product  Inputs=*/  OutDataTypeStr=Inherit: Inherit via back propagation
  Sum : Sum  OutDataTypeStr=Inherit: Inherit via back propagation  RndMeth=Zero
  GcDAS_CellMaxTempTi1_min : Outport
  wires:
  Data Store Read/1 -> Sum/1
  Constant10/1 -> Data Type Conversion/1
  Data Type Conversion/1 -> Product1/1
  Product1/1 -> Sum/2
  Constant1/1 -> Data Type Conversion1/1
  Data Type Conversion1/1 -> Product1/2
  Sum/1 -> Limiter/3
  Limiter/1 -> OverWrite/1
  Constant2/1 -> Limiter/2
  Constant3/1 -> Limiter/1
  OverWrite/1 -> Data Store Write/1, GcDAS_CellMaxTempTi1_min/1  "GcDAS_CellMaxTempTi1_min"

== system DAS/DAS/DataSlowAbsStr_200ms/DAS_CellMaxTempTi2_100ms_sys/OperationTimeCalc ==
  Enable : EnablePort
  Constant1 : Constant  Value=DAS_MIN2MS_NUMB
  Constant10 : Constant  Value=DAS_RUNTIME100_MS
  Constant2 : Constant  Value=DAS_STATSTIMEMIN_MIN
  Constant3 : Constant  Value=DAS_STATSTIMEMAX_MIN
  Data Store Read : AIWAYS_Powertrain_BMS_lib/Signals/Data Store Read  Priority=0  DSR=EcNVM_CellMaxTempTi2_min
  Data Store Write : AIWAYS_Powertrain_BMS_lib/Signals/Data Store Write  DSW=EcNVM_CellMaxTempTi2_min
  Data Type Conversion : DataTypeConversion  OutDataTypeStr=single
  Data Type Conversion1 : DataTypeConversion  OutDataTypeStr=single
  Limiter : AIWAYS_Powertrain_BMS_lib/Nonlinear Blocks/Limiter
  OverWrite : AIWAYS_Powertrain_BMS_lib/Signals/OverWrite  OverWrite_Value=CcDAS_CellMaxTempTi2Ovr_min  OverWrite_flag=CbDAS_CellMaxTempTi2OvrSwt_flg
  Product1 : Product  Inputs=*/  OutDataTypeStr=Inherit: Inherit via back propagation
  Sum : Sum  OutDataTypeStr=Inherit: Inherit via back propagation  RndMeth=Zero
  GcDAS_CellMaxTempTi2_min : Outport
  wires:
  Data Store Read/1 -> Sum/1
  Constant10/1 -> Data Type Conversion/1
  Data Type Conversion/1 -> Product1/1
  Product1/1 -> Sum/2
  Constant1/1 -> Data Type Conversion1/1
  Data Type Conversion1/1 -> Product1/2
  Sum/1 -> Limiter/3
  Limiter/1 -> OverWrite/1
  Constant2/1 -> Limiter/2
  Constant3/1 -> Limiter/1
  OverWrite/1 -> Data Store Write/1, GcDAS_CellMaxTempTi2_min/1  "GcDAS_CellMaxTempTi2_min"

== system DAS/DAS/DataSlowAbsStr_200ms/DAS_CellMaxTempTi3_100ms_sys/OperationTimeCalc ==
  Enable : EnablePort
  Constant1 : Constant  Value=DAS_MIN2MS_NUMB
  Constant10 : Constant  Value=DAS_RUNTIME100_MS
  Constant2 : Constant  Value=DAS_STATSTIMEMIN_MIN
  Constant3 : Constant  Value=DAS_STATSTIMEMAX_MIN
  Data Store Read : AIWAYS_Powertrain_BMS_lib/Signals/Data Store Read  Priority=0  DSR=EcNVM_CellMaxTempTi3_min
  Data Store Write : AIWAYS_Powertrain_BMS_lib/Signals/Data Store Write  DSW=EcNVM_CellMaxTempTi3_min
  Data Type Conversion : DataTypeConversion  OutDataTypeStr=single
  Data Type Conversion1 : DataTypeConversion  OutDataTypeStr=single
  Limiter : AIWAYS_Powertrain_BMS_lib/Nonlinear Blocks/Limiter
  OverWrite : AIWAYS_Powertrain_BMS_lib/Signals/OverWrite  OverWrite_Value=CcDAS_CellMaxTempTi3Ovr_min  OverWrite_flag=CbDAS_CellMaxTempTi3OvrSwt_flg
  Product1 : Product  Inputs=*/  OutDataTypeStr=Inherit: Inherit via back propagation
  Sum : Sum  OutDataTypeStr=Inherit: Inherit via back propagation  RndMeth=Zero
  GcDAS_CellMaxTempTi3_min : Outport
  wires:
  Data Store Read/1 -> Sum/1
  Constant10/1 -> Data Type Conversion/1
  Data Type Conversion/1 -> Product1/1
  Product1/1 -> Sum/2
  Constant1/1 -> Data Type Conversion1/1
  Data Type Conversion1/1 -> Product1/2
  Sum/1 -> Limiter/3
  Limiter/1 -> OverWrite/1
  Constant2/1 -> Limiter/2
  Constant3/1 -> Limiter/1
  OverWrite/1 -> Data Store Write/1, GcDAS_CellMaxTempTi3_min/1  "GcDAS_CellMaxTempTi3_min"

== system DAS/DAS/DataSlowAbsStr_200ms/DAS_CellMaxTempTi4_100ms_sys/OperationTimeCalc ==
  Enable : EnablePort
  Constant1 : Constant  Value=DAS_MIN2MS_NUMB
  Constant10 : Constant  Value=DAS_RUNTIME100_MS
  Constant2 : Constant  Value=DAS_STATSTIMEMIN_MIN
  Constant3 : Constant  Value=DAS_STATSTIMEMAX_MIN
  Data Store Read : AIWAYS_Powertrain_BMS_lib/Signals/Data Store Read  Priority=0  DSR=EcNVM_CellMaxTempTi4_min
  Data Store Write : AIWAYS_Powertrain_BMS_lib/Signals/Data Store Write  DSW=EcNVM_CellMaxTempTi4_min
  Data Type Conversion : DataTypeConversion  OutDataTypeStr=single
  Data Type Conversion1 : DataTypeConversion  OutDataTypeStr=single
  Limiter : AIWAYS_Powertrain_BMS_lib/Nonlinear Blocks/Limiter
  OverWrite : AIWAYS_Powertrain_BMS_lib/Signals/OverWrite  OverWrite_Value=CcDAS_CellMaxTempTi4Ovr_min  OverWrite_flag=CbDAS_CellMaxTempTi4OvrSwt_flg
  Product1 : Product  Inputs=*/  OutDataTypeStr=Inherit: Inherit via back propagation
  Sum : Sum  OutDataTypeStr=Inherit: Inherit via back propagation  RndMeth=Zero
  GcDAS_CellMaxTempTi4_min : Outport
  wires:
  Data Store Read/1 -> Sum/1
  Constant10/1 -> Data Type Conversion/1
  Data Type Conversion/1 -> Product1/1
  Product1/1 -> Sum/2
  Constant1/1 -> Data Type Conversion1/1
  Data Type Conversion1/1 -> Product1/2
  Sum/1 -> Limiter/3
  Limiter/1 -> OverWrite/1
  Constant2/1 -> Limiter/2
  Constant3/1 -> Limiter/1
  OverWrite/1 -> Data Store Write/1, GcDAS_CellMaxTempTi4_min/1  "GcDAS_CellMaxTempTi4_min"

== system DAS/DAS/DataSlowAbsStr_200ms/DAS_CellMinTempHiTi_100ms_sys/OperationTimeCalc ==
  Enable : EnablePort
  Constant1 : Constant  Value=DAS_MIN2MS_NUMB
  Constant10 : Constant  Value=DAS_RUNTIME100_MS
  Constant2 : Constant  Value=DAS_STATSTIMEMIN_MIN
  Constant3 : Constant  Value=DAS_STATSTIMEMAX_MIN
  Data Store Read : AIWAYS_Powertrain_BMS_lib/Signals/Data Store Read  Priority=0  DSR=EcNVM_CellMinTempHiTi_min
  Data Store Write : AIWAYS_Powertrain_BMS_lib/Signals/Data Store Write  DSW=EcNVM_CellMinTempHiTi_min
  Data Type Conversion : DataTypeConversion  OutDataTypeStr=single
  Data Type Conversion1 : DataTypeConversion  OutDataTypeStr=single
  Limiter : AIWAYS_Powertrain_BMS_lib/Nonlinear Blocks/Limiter
  OverWrite : AIWAYS_Powertrain_BMS_lib/Signals/OverWrite  OverWrite_Value=CcDAS_MinTempHiTiOvr_min  OverWrite_flag=CbDAS_MinTempHiTiOvrSwt_flg
  Product1 : Product  Inputs=*/  OutDataTypeStr=Inherit: Inherit via back propagation
  Sum : Sum  OutDataTypeStr=Inherit: Inherit via back propagation  RndMeth=Zero
  GcDAS_CellMinTempHiTi_min : Outport
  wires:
  Data Store Read/1 -> Sum/1
  Constant10/1 -> Data Type Conversion/1
  Data Type Conversion/1 -> Product1/1
  Product1/1 -> Sum/2
  Constant1/1 -> Data Type Conversion1/1
  Data Type Conversion1/1 -> Product1/2
  Sum/1 -> Limiter/3
  Limiter/1 -> OverWrite/1
  Constant2/1 -> Limiter/2
  Constant3/1 -> Limiter/1
  OverWrite/1 -> Data Store Write/1, GcDAS_CellMinTempHiTi_min/1  "GcDAS_CellMinTempHiTi_min"

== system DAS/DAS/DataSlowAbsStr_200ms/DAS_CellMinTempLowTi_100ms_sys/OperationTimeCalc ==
  Enable : EnablePort
  Constant1 : Constant  Value=DAS_MIN2MS_NUMB
  Constant10 : Constant  Value=DAS_RUNTIME100_MS
  Constant2 : Constant  Value=DAS_STATSTIMEMIN_MIN
  Constant3 : Constant  Value=DAS_STATSTIMEMAX_MIN
  Data Store Read : AIWAYS_Powertrain_BMS_lib/Signals/Data Store Read  Priority=0  DSR=EcNVM_CellMinTempLowTi_min
  Data Store Write : AIWAYS_Powertrain_BMS_lib/Signals/Data Store Write  DSW=EcNVM_CellMinTempLowTi_min
  Data Type Conversion : DataTypeConversion  OutDataTypeStr=single
  Data Type Conversion1 : DataTypeConversion  OutDataTypeStr=single
  Limiter : AIWAYS_Powertrain_BMS_lib/Nonlinear Blocks/Limiter
  OverWrite : AIWAYS_Powertrain_BMS_lib/Signals/OverWrite  OverWrite_Value=CcDAS_MinTempLowTiOvr_min  OverWrite_flag=CbDAS_MinTempLowTiOvrSwt_flg
  Product1 : Product  Inputs=*/  OutDataTypeStr=Inherit: Inherit via back propagation
  Sum : Sum  OutDataTypeStr=Inherit: Inherit via back propagation  RndMeth=Zero
  GcDAS_CellMinTempLowTi_min : Outport
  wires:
  Data Store Read/1 -> Sum/1
  Constant10/1 -> Data Type Conversion/1
  Data Type Conversion/1 -> Product1/1
  Product1/1 -> Sum/2
  Constant1/1 -> Data Type Conversion1/1
  Data Type Conversion1/1 -> Product1/2
  Sum/1 -> Limiter/3
  Limiter/1 -> OverWrite/1
  Constant2/1 -> Limiter/2
  Constant3/1 -> Limiter/1
  OverWrite/1 -> Data Store Write/1, GcDAS_CellMinTempLowTi_min/1  "GcDAS_CellMinTempLowTi_min"

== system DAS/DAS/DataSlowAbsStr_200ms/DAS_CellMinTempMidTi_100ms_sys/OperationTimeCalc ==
  Enable : EnablePort
  Constant1 : Constant  Value=DAS_MIN2MS_NUMB
  Constant10 : Constant  Value=DAS_RUNTIME100_MS
  Constant2 : Constant  Value=DAS_STATSTIMEMIN_MIN
  Constant3 : Constant  Value=DAS_STATSTIMEMAX_MIN
  Data Store Read : AIWAYS_Powertrain_BMS_lib/Signals/Data Store Read  Priority=0  DSR=EcNVM_CellMinTempMidTi_min
  Data Store Write : AIWAYS_Powertrain_BMS_lib/Signals/Data Store Write  DSW=EcNVM_CellMinTempMidTi_min
  Data Type Conversion : DataTypeConversion  OutDataTypeStr=single
  Data Type Conversion1 : DataTypeConversion  OutDataTypeStr=single
  Limiter : AIWAYS_Powertrain_BMS_lib/Nonlinear Blocks/Limiter
  OverWrite : AIWAYS_Powertrain_BMS_lib/Signals/OverWrite  OverWrite_Value=CcDAS_MinTempMidTiOvr_min  OverWrite_flag=CbDAS_MinTempMidTiOvrSwt_flg
  Product1 : Product  Inputs=*/  OutDataTypeStr=Inherit: Inherit via back propagation
  Sum : Sum  OutDataTypeStr=Inherit: Inherit via back propagation  RndMeth=Zero
  GcDAS_CellMinTempMidTi_min : Outport
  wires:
  OverWrite/1 -> Data Store Write/1, GcDAS_CellMinTempMidTi_min/1  "GcDAS_CellMinTempMidTi_min"
  Constant3/1 -> Limiter/1
  Constant2/1 -> Limiter/2
  Limiter/1 -> OverWrite/1
  Sum/1 -> Limiter/3
  Data Type Conversion1/1 -> Product1/2
  Constant1/1 -> Data Type Conversion1/1
  Product1/1 -> Sum/2
  Data Type Conversion/1 -> Product1/1
  Constant10/1 -> Data Type Conversion/1
  Data Store Read/1 -> Sum/1

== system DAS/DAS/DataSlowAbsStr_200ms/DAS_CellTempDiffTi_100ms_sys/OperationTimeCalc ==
  Enable : EnablePort
  Constant1 : Constant  Value=DAS_MIN2MS_NUMB
  Constant10 : Constant  Value=DAS_RUNTIME100_MS
  Constant2 : Constant  Value=DAS_STATSTIMEMIN_MIN
  Constant3 : Constant  Value=DAS_STATSTIMEMAX_MIN
  Data Store Read : AIWAYS_Powertrain_BMS_lib/Signals/Data Store Read  Priority=0  DSR=EcNVM_CellTempDiffLimTi_min
  Data Store Write : AIWAYS_Powertrain_BMS_lib/Signals/Data Store Write  DSW=EcNVM_CellTempDiffLimTi_min
  Data Type Conversion : DataTypeConversion  OutDataTypeStr=single
  Data Type Conversion1 : DataTypeConversion  OutDataTypeStr=single
  Limiter : AIWAYS_Powertrain_BMS_lib/Nonlinear Blocks/Limiter
  OverWrite : AIWAYS_Powertrain_BMS_lib/Signals/OverWrite  OverWrite_Value=CcDAS_CellTempDiffLimTiOvr_min  OverWrite_flag=CbDAS_CellTempDiffLimTiOvrSwt_flg
  Product1 : Product  Inputs=*/  OutDataTypeStr=Inherit: Inherit via back propagation
  Sum : Sum  OutDataTypeStr=Inherit: Inherit via back propagation  RndMeth=Zero
  GcDAS_CellTempDiffLimTi_min : Outport
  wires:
  Data Store Read/1 -> Sum/1
  Constant10/1 -> Data Type Conversion/1
  Data Type Conversion/1 -> Product1/1
  Product1/1 -> Sum/2
  Constant1/1 -> Data Type Conversion1/1
  Data Type Conversion1/1 -> Product1/2
  Sum/1 -> Limiter/3
  Limiter/1 -> OverWrite/1
  Constant2/1 -> Limiter/2
  Constant3/1 -> Limiter/1
  OverWrite/1 -> Data Store Write/1, GcDAS_CellTempDiffLimTi_min/1  "GcDAS_CellTempDiffLimTi_min"

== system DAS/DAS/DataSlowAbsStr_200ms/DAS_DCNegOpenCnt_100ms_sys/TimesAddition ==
  Enable : EnablePort
  ACC_GbACC_ACChrgMismatch_flg : AIWAYS_Powertrain_BMS_lib/Signals/OverWrite  OverWrite_Value=CcDAS_DCNegOpenCntOvr_numb  OverWrite_flag=CbDAS_DCNegOpenCntOvrSwt_flg
  Constant : Constant  Value=DAS_TIMESONE_NUMB
  Constant4 : Constant  Value=DAS_STATSTIMESMIN_NUMB
  Constant5 : Constant  Value=DAS_STATSTIMESMAX_NUMB
  Data Store Read : AIWAYS_Powertrain_BMS_lib/Signals/Data Store Read  Priority=0  DSR=EcNVM_DCNegOpenCnt_numb
  Data Store Write : AIWAYS_Powertrain_BMS_lib/Signals/Data Store Write  DSW=EcNVM_DCNegOpenCnt_numb
  Limiter : AIWAYS_Powertrain_BMS_lib/Nonlinear Blocks/Limiter
  Sum : Sum  OutDataTypeStr=Inherit: Inherit via back propagation  RndMeth=Zero
  GcDAS_DCNegOpenCnt_numb : Outport
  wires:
  Data Store Read/1 -> Sum/1
  Sum/1 -> Limiter/3
  ACC_GbACC_ACChrgMismatch_flg/1 -> GcDAS_DCNegOpenCnt_numb/1, Data Store Write/1  "GcDAS_DCNegOpenCnt_numb"
  Constant/1 -> Sum/2
  Constant5/1 -> Limiter/1
  Constant4/1 -> Limiter/2
  Limiter/1 -> ACC_GbACC_ACChrgMismatch_flg/1

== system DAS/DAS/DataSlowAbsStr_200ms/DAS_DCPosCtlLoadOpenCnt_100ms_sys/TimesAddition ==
  Enable : EnablePort
  ACC_GbACC_ACChrgMismatch_flg : AIWAYS_Powertrain_BMS_lib/Signals/OverWrite  OverWrite_Value=CcDAS_DCPosCtlLoadOpenCntOvr_numb  OverWrite_flag=CbDAS_DCPosCtlLoadOpenCntOvrSwt_flg
  Constant : Constant  Value=DAS_TIMESONE_NUMB
  Constant4 : Constant  Value=DAS_STATSTIMESMIN_NUMB
  Constant5 : Constant  Value=DAS_STATSTIMESMAX_NUMB
  Data Store Read : AIWAYS_Powertrain_BMS_lib/Signals/Data Store Read  Priority=0  DSR=EcNVM_DCPosCtlLoadOpenCnt_numb
  Data Store Write : AIWAYS_Powertrain_BMS_lib/Signals/Data Store Write  DSW=EcNVM_DCPosCtlLoadOpenCnt_numb
  Limiter : AIWAYS_Powertrain_BMS_lib/Nonlinear Blocks/Limiter
  Sum : Sum  OutDataTypeStr=Inherit: Inherit via back propagation  RndMeth=Zero
  GcDAS_DCPosCtlLoadOpenCnt_numb : Outport
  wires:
  Data Store Read/1 -> Sum/1
  Sum/1 -> Limiter/3
  ACC_GbACC_ACChrgMismatch_flg/1 -> GcDAS_DCPosCtlLoadOpenCnt_numb/1, Data Store Write/1  "GcDAS_DCPosCtlLoadOpenCnt_numb"
  Constant/1 -> Sum/2
  Constant5/1 -> Limiter/1
  Constant4/1 -> Limiter/2
  Limiter/1 -> ACC_GbACC_ACChrgMismatch_flg/1

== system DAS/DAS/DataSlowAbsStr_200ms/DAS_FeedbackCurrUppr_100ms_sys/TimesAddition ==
  Enable : EnablePort
  ACC_GbACC_ACChrgMismatch_flg : AIWAYS_Powertrain_BMS_lib/Signals/OverWrite  OverWrite_Value=CcDAS_FeedbackCurrUpprLimCntOvr_numb  OverWrite_flag=CbDAS_FeedbackCurrUpprLimCntOvrSwt_flg
  Constant : Constant  Value=DAS_TIMESONE_NUMB
  Constant4 : Constant  Value=DAS_STATSTIMESMIN_NUMB
  Constant5 : Constant  Value=DAS_STATSTIMESMAX_NUMB
  Data Store Read : AIWAYS_Powertrain_BMS_lib/Signals/Data Store Read  Priority=0  DSR=EcNVM_FeedbackCurrUpprLimCnt_numb
  Data Store Write : AIWAYS_Powertrain_BMS_lib/Signals/Data Store Write  DSW=EcNVM_FeedbackCurrUpprLimCnt_numb
  Limiter : AIWAYS_Powertrain_BMS_lib/Nonlinear Blocks/Limiter
  Sum : Sum  OutDataTypeStr=Inherit: Inherit via back propagation  RndMeth=Zero
  GcDAS_FeedbackCurrUpprLimCnt_numb : Outport
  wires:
  Data Store Read/1 -> Sum/1
  Sum/1 -> Limiter/3
  ACC_GbACC_ACChrgMismatch_flg/1 -> GcDAS_FeedbackCurrUpprLimCnt_numb/1, Data Store Write/1  "GcDAS_FeedbackCurrUpprLimCnt_numb"
  Constant/1 -> Sum/2
  Constant5/1 -> Limiter/1
  Constant4/1 -> Limiter/2
  Limiter/1 -> ACC_GbACC_ACChrgMismatch_flg/1

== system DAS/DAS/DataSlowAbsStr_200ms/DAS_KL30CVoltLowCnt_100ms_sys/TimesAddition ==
  Enable : EnablePort
  ACC_GbACC_ACChrgMismatch_flg : AIWAYS_Powertrain_BMS_lib/Signals/OverWrite  OverWrite_Value=CcDAS_KL30CVoltLowCntOvr_numb  OverWrite_flag=CbDAS_KL30CVoltLowCntOvrSwt_flg
  Constant : Constant  Value=DAS_TIMESONE_NUMB
  Constant1 : Constant  Value=DAS_STATSTIMESMAX_NUMB
  Constant2 : Constant  Value=DAS_STATSTIMESMIN_NUMB
  Data Store Read : AIWAYS_Powertrain_BMS_lib/Signals/Data Store Read  Priority=0  DSR=EcNVM_KL30CVoltLowCnt_numb
  Data Store Write : AIWAYS_Powertrain_BMS_lib/Signals/Data Store Write  DSW=EcNVM_KL30CVoltLowCnt_numb
  Data Type Conversion : DataTypeConversion  OutDataTypeStr=uint16
  Limiter : AIWAYS_Powertrain_BMS_lib/Nonlinear Blocks/Limiter
  Sum : Sum  OutDataTypeStr=Inherit: Inherit via back propagation  RndMeth=Zero
  GcDAS_KL30CVoltLowCnt_numb : Outport
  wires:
  Data Store Read/1 -> Sum/1
  ACC_GbACC_ACChrgMismatch_flg/1 -> Data Store Write/1, GcDAS_KL30CVoltLowCnt_numb/1  "GcDAS_KL30CVoltLowCnt_numb"
  Constant/1 -> Data Type Conversion/1
  Limiter/1 -> ACC_GbACC_ACChrgMismatch_flg/1
  Sum/1 -> Limiter/3
  Constant1/1 -> Limiter/1
  Constant2/1 -> Limiter/2
  Data Type Conversion/1 -> Sum/2

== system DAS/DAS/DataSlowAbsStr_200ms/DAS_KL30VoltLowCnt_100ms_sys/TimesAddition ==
  Enable : EnablePort
  ACC_GbACC_ACChrgMismatch_flg : AIWAYS_Powertrain_BMS_lib/Signals/OverWrite  OverWrite_Value=CcDAS_KL30VoltLowCntOvr_numb  OverWrite_flag=CbDAS_KL30VoltLowCntOvrSwt_flg
  Constant : Constant  Value=DAS_TIMESONE_NUMB
  Constant1 : Constant  Value=DAS_STATSTIMESMAX_NUMB
  Constant2 : Constant  Value=DAS_STATSTIMESMIN_NUMB
  Data Store Read : AIWAYS_Powertrain_BMS_lib/Signals/Data Store Read  Priority=0  DSR=EcNVM_KL30VoltLowCnt_numb
  Data Store Write : AIWAYS_Powertrain_BMS_lib/Signals/Data Store Write  DSW=EcNVM_KL30VoltLowCnt_numb
  Data Type Conversion : DataTypeConversion  OutDataTypeStr=uint16
  Limiter : AIWAYS_Powertrain_BMS_lib/Nonlinear Blocks/Limiter
  Sum : Sum  OutDataTypeStr=Inherit: Inherit via back propagation  RndMeth=Zero
  GcDAS_KL30VoltLowCnt_numb : Outport
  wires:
  Data Store Read/1 -> Sum/1
  ACC_GbACC_ACChrgMismatch_flg/1 -> Data Store Write/1, GcDAS_KL30VoltLowCnt_numb/1  "GcDAS_KL30VoltLowCnt_numb"
  Constant/1 -> Data Type Conversion/1
  Limiter/1 -> ACC_GbACC_ACChrgMismatch_flg/1
  Sum/1 -> Limiter/3
  Constant1/1 -> Limiter/1
  Constant2/1 -> Limiter/2
  Data Type Conversion/1 -> Sum/2

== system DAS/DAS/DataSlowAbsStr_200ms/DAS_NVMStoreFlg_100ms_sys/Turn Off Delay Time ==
  note: Turn Off Delay Time
  T : Inport
  u : Inport  Port=2
  dT : Inport  Port=3
  AND : Logic  Operator=OR  OutDataTypeStr=boolean
  Constant Value1 : Constant  Value=0  OutDataTypeStr=Inherit: Inherit via back propagation
  Constant Value2 : Constant  Value=0  OutDataTypeStr=Inherit: Inherit via back propagation
  EdgeFalling1 : Subsystem  Tag=R11-1  TreatAsAtomicUnit=on  mask(EdgeFalling){}
      mask help: The output indicates true if the logical input value changes from true to false. Input1=Value (u).
  Greater Than : RelationalOperator  Operator=>  OutDataTypeStr=boolean
  Minimum : MinMax  Function=max  Inputs=2
  Summation : Sum  Inputs=-+
  Switch : Switch  Criteria=u2 ~= 0  Threshold=1  RndMeth=Zero
  Unit Delay : UnitDelay  SampleTime=-1
  y : Outport
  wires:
  T/1 -> Switch/1
  EdgeFalling1/1(y) -> Switch/2
  Constant Value1/1 -> Minimum/2
  Summation/1 -> Minimum/1
  Constant Value2/1 -> Greater Than/2
  Unit Delay/1 -> Summation/2
  u/1 -> EdgeFalling1/1(u), AND/1
  AND/1 -> y/1
  Greater Than/1 -> AND/2
  Switch/1 -> Greater Than/1, Unit Delay/1
  dT/1 -> Summation/1
  Minimum/1 -> Switch/3

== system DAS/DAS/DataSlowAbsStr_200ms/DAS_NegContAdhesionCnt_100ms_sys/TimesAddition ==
  Enable : EnablePort
  ACC_GbACC_ACChrgMismatch_flg : AIWAYS_Powertrain_BMS_lib/Signals/OverWrite  OverWrite_Value=CcDAS_NegContAdhesionCntOvr_numb  OverWrite_flag=CbDAS_NegContAdhesionCntOvrSwt_flg
  Constant : Constant  Value=DAS_TIMESONE_NUMB
  Constant4 : Constant  Value=DAS_STATSTIMESMIN_NUMB
  Constant5 : Constant  Value=DAS_STATSTIMESMAX_NUMB
  Data Store Read : AIWAYS_Powertrain_BMS_lib/Signals/Data Store Read  Priority=0  DSR=EcNVM_NegContAdhesionCnt_numb
  Data Store Write : AIWAYS_Powertrain_BMS_lib/Signals/Data Store Write  DSW=EcNVM_NegContAdhesionCnt_numb
  Limiter : AIWAYS_Powertrain_BMS_lib/Nonlinear Blocks/Limiter
  Sum : Sum  OutDataTypeStr=Inherit: Inherit via back propagation  RndMeth=Zero
  GcDAS_NegContAdhesionCnt_numb : Outport
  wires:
  Data Store Read/1 -> Sum/1
  Sum/1 -> Limiter/3
  ACC_GbACC_ACChrgMismatch_flg/1 -> GcDAS_NegContAdhesionCnt_numb/1, Data Store Write/1  "GcDAS_NegContAdhesionCnt_numb"
  Constant/1 -> Sum/2
  Constant5/1 -> Limiter/1
  Constant4/1 -> Limiter/2
  Limiter/1 -> ACC_GbACC_ACChrgMismatch_flg/1

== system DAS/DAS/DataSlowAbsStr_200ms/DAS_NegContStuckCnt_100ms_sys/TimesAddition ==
  Enable : EnablePort
  ACC_GbACC_ACChrgMismatch_flg : AIWAYS_Powertrain_BMS_lib/Signals/OverWrite  OverWrite_Value=CcDAS_NegContStuckCntOvr_numb  OverWrite_flag=CbDAS_NegContStuckCntOvrSwt_flg
  Constant : Constant  Value=DAS_TIMESONE_NUMB
  Constant4 : Constant  Value=DAS_STATSTIMESMIN_NUMB
  Constant5 : Constant  Value=DAS_STATSTIMESMAX_NUMB
  Data Store Read : AIWAYS_Powertrain_BMS_lib/Signals/Data Store Read  Priority=0  DSR=EcNVM_NegContStuckCnt_numb
  Data Store Write : AIWAYS_Powertrain_BMS_lib/Signals/Data Store Write  DSW=EcNVM_NegContStuckCnt_numb
  Limiter : AIWAYS_Powertrain_BMS_lib/Nonlinear Blocks/Limiter
  Sum : Sum  OutDataTypeStr=Inherit: Inherit via back propagation  RndMeth=Zero
  GcDAS_NegContStuckCnt_numb : Outport
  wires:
  Data Store Read/1 -> Sum/1
  Sum/1 -> Limiter/3
  ACC_GbACC_ACChrgMismatch_flg/1 -> GcDAS_NegContStuckCnt_numb/1, Data Store Write/1  "GcDAS_NegContStuckCnt_numb"
  Constant/1 -> Sum/2
  Constant5/1 -> Limiter/1
  Constant4/1 -> Limiter/2
  Limiter/1 -> ACC_GbACC_ACChrgMismatch_flg/1
